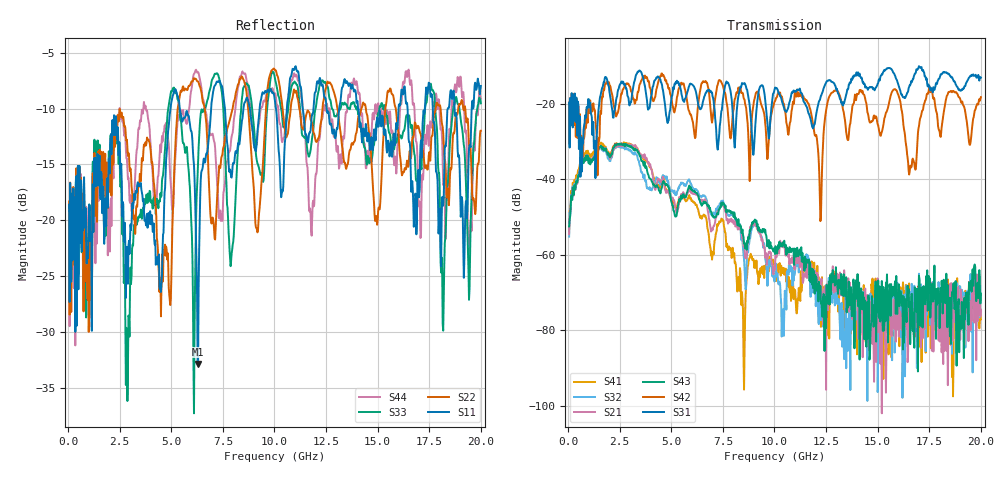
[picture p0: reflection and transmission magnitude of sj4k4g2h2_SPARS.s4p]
! FILE: E:\users\goganessyan\GBX_Backplane\FR408_backplane\1m_INBOUND_FEXT\sj4k4g2h2_SPARS.s4p
# MHZ S RI R 50.00
! FREQ  S11  S12  S13  S14
!  S21  S22  S23  S24
!  S31  S32  S33  S34
!  S41  S42  S43  S44
!  REAL  IMAG  REAL  IMAG  REAL  IMAG  REAL  IMAG
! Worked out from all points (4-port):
!   799 points, 50 MHz to 20 GHz, reference 50 ohm
!   strongest paths, dB at 50 MHz, 5.025 GHz, 10.03 GHz, 15.03 GHz, 20 GHz:
!     S31: -19.7, -18.0, -15.8, -14.5, -13.1
!     S42: -19.7, -19.3, -19.4, -25.7, -18.3
!     S43: -52.5, -46.3, -59.8, -66.8, -70.3
!     S21: -54.6, -44.9, -63.1, -80.5, -74.6
!     S32: -55.2, -42.9, -65.9, -85.1, -72.1
!     S41: -53.4, -45.7, -63.5, -72.6, -77.1
!   lowest |S11| = -32.9 dB at 6.3 GHz (marker M1), VSWR 1.05, Z = 48.3 - j1.46 ohm
!   |S11| at or under -10 dB: start of sweep to 4.964 GHz; 5.413 GHz to 6.929 GHz (1.516 GHz wide, 24.6 % of centre); 14.05 GHz to 16.01 GHz (1.965 GHz wide, 13.1 % of centre)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
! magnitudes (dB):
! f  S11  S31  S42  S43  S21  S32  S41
! 50 MHz  -18.6  -19.7  -19.7  -52.5  -54.6  -55.2  -53.4
! 1.55 GHz  -16.6  -18.2  -23.0  -31.3  -31.5  -31.6  -30.5
! 6.3 GHz  -32.9  -20.0  -20.3  -44.3  -44.6  -43.3  -48.0
! 8.5 GHz  -9.9  -14.7  -18.4  -55.3  -57.6  -60.0  -86.7
! 12.22 GHz  -7.4  -18.4  -51.1  -68.3  -67.4  -73.3  -67.7
! 12.9 GHz  -12.2  -14.7  -16.5  -65.6  -66.1  -67.7  -66.0
! 20 GHz  -8.0  -13.1  -18.3  -70.3  -74.6  -72.1  -77.1
